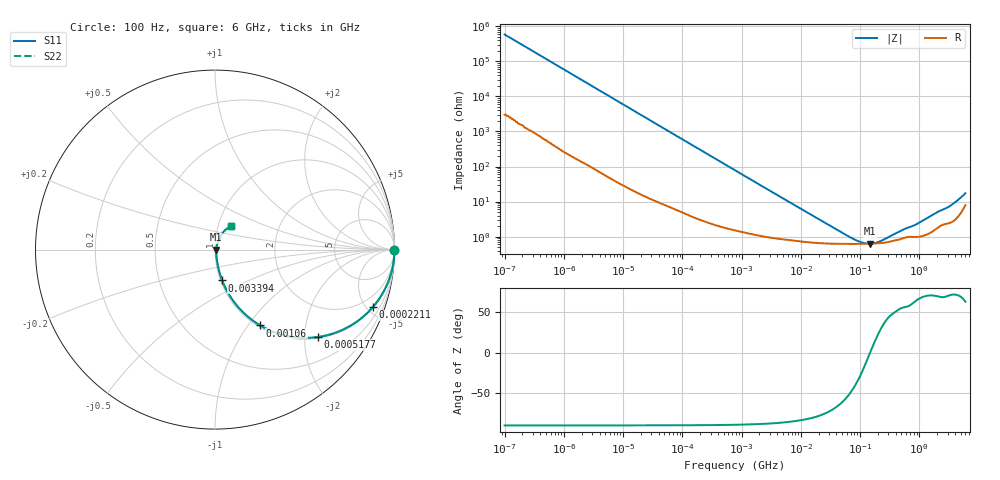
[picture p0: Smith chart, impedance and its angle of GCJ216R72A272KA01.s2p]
!Murata Part Number: GCJ216R72A272KA01
!These Parameters are Measured in Series Mode Connection
!Data Generated on Mar 13, 2026
!  o--ll--o
!Port1  Port2
!  o------o
!Operation Temp=25[degC], DC Bias Voltage=0[V]
!Freq. Start=100[Hz] Stop=6[GHz] 401[Steps]
# Hz S RI R 50
!Freq.(Hz) S11(Real) S11(Imag) S21(Real) S21(Imag) S12(Real) S12(Imag) S22(Real) S22(Imag)
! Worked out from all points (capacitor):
!   401 points, 100 Hz to 6 GHz, reference 50 ohm
!   read as one part in series: C = 2.71 nF near 109 Hz
!   lowest |Z| = 629 mohm at 145.9 MHz (marker M1)
!   series resonance near 148 MHz, so ESL is about 430 pH
!   S11 on the Smith chart (normalised r, x): 100 Hz: open; 221.1 kHz: 1.06, -5.44; 517.7 kHz: 1.04, -2.33; 1.06 MHz: 1.03, -1.14; 3.394 MHz: 1.02, -0.36; 6 GHz: 1.16, +0.31
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100  1 -0.000171  9e-07 0.000171  9e-07 0.000171  1 -0.000171
2008  1 -0.0034  2.71e-05 0.0034  2.71e-05 0.0034  1 -0.0034
40335  0.995 -0.0673  0.00497 0.0673  0.00497 0.0673  0.995 -0.0673
98762  0.9723 -0.1602  0.0277 0.1602  0.0277 0.1602  0.9723 -0.1602
221108  0.8782 -0.3219  0.1218 0.3219  0.1218 0.3219  0.8782 -0.3219
330837  0.7654 -0.4177  0.2346 0.4177  0.2346 0.4177  0.7654 -0.4177
517687  0.575 -0.4868  0.425 0.4868  0.425 0.4868  0.575 -0.4868
774597  0.3811 -0.4761  0.6189 0.4761  0.6189 0.4761  0.3811 -0.4761
1059725  0.2517 -0.4225  0.7483 0.4225  0.7483 0.4225  0.2517 -0.4225
1813585  0.1092 -0.296  0.8908 0.296  0.8908 0.296  0.1092 -0.296
3394479  0.0397 -0.1717  0.9603 0.1717  0.9603 0.1717  0.0397 -0.1717
6644369  0.0162 -0.0907  0.9838 0.0907  0.9838 0.0907  0.0162 -0.0907
1.555665e7  0.00826 -0.0393  0.9917 0.0393  0.9917 0.0393  0.00826 -0.0393
7.797396e7  0.00619 -0.00579  0.9938 0.00579  0.9938 0.00579  0.00619 -0.00579
1.115611e8  0.00619 -0.00242  0.9938 0.00242  0.9938 0.00242  0.00619 -0.00242
1.459435e8  0.00625 -0.000114  0.9937 0.000114  0.9937 0.000114  0.00625 -0.000114
1.996653e8  0.00642 0.00258  0.9936 -0.00258  0.9936 -0.00258  0.00642 0.00258
3.124326e8  0.00713 0.00691  0.9929 -0.00691  0.9929 -0.00691  0.00713 0.00691
8.749838e8  0.01 0.0195  0.99 -0.0195  0.99 -0.0195  0.01 0.0195
1.873145e9  0.0176 0.0426  0.9824 -0.0426  0.9824 -0.0426  0.0176 0.0426
3.065283e9  0.0271 0.0623  0.9729 -0.0623  0.9729 -0.0623  0.0271 0.0623
6e9  0.0918 0.1292  0.9082 -0.1292  0.9082 -0.1292  0.0918 0.1292
